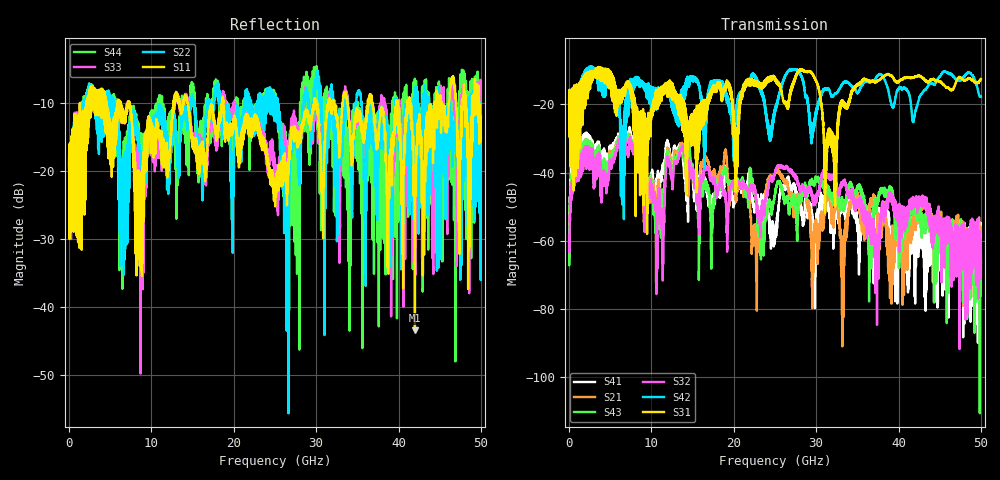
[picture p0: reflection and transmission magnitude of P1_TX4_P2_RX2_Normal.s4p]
!Keysight Technologies,N5225B,MY57041031,A.13.20.10
!Date: Friday, May 31, 2019 11:30:07
!Correction: S11(Full 4 Port(1,2,3,4))
!S12(Full 4 Port(1,2,3,4))
!S13(Full 4 Port(1,2,3,4))
!S14(Full 4 Port(1,2,3,4))
!S21(Full 4 Port(1,2,3,4))
!S22(Full 4 Port(1,2,3,4))
!S23(Full 4 Port(1,2,3,4))
!S24(Full 4 Port(1,2,3,4))
!S31(Full 4 Port(1,2,3,4))
!S32(Full 4 Port(1,2,3,4))
!S33(Full 4 Port(1,2,3,4))
!S34(Full 4 Port(1,2,3,4))
!S41(Full 4 Port(1,2,3,4))
!S42(Full 4 Port(1,2,3,4))
!S43(Full 4 Port(1,2,3,4))
!S44(Full 4 Port(1,2,3,4))
!S4P File: Measurements: <S11,S12,S13,S14>,
!<S21,S22,S23,S24>,
!<S31,S32,S33,S34>,
!<S41,S42,S43,S44>:
# Hz S  dB  R 50.0
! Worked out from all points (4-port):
!   5000 points, 10 MHz to 50 GHz, reference 50 ohm
!   strongest paths, dB at 10 MHz, 12.51 GHz, 25.01 GHz, 37.51 GHz, 50 GHz:
!     S31: -19.6, -17.9, -13.0, -13.1, -12.6
!     S42: -19.5, -15.9, -21.5, -11.4, -17.7
!     S32: -60.1, -41.7, -39.9, -62.8, -66.4
!     S43: -62.0, -40.3, -46.1, -48.8, -66.5
!     S21: -61.4, -38.6, -40.4, -55.7, -68.5
!     S41: -58.4, -35.8, -58.5, -51.1, -70.3
!   lowest |S11| = -43.4 dB at 41.99 GHz (marker M1), VSWR 1.01, Z = 50.7 - j0.157 ohm
!   |S11| at or under -10 dB: 7.334 GHz to 12.7 GHz (5.363 GHz wide, 53.5 % of centre); 14.44 GHz to 18.57 GHz (4.131 GHz wide, 25 % of centre); 18.74 GHz to 29.76 GHz (11.02 GHz wide, 45.4 % of centre)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
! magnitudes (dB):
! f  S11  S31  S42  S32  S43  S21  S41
! 10 MHz  -19.5  -19.6  -19.5  -60.1  -62.0  -61.4  -58.4
! 7.05 GHz  -11.0  -14.7  -22.4  -33.1  -29.1  -30.6  -28.9
! 10.47 GHz  -17.1  -17.5  -15.4  -48.0  -51.9  -52.2  -47.8
! 29.22 GHz  -12.6  -10.3  -25.2  -44.5  -43.0  -53.7  -50.9
! 32.24 GHz  -10.5  -35.9  -17.0  -42.5  -47.9  -51.3  -57.6
! 41.99 GHz  -43.4  -11.9  -22.7  -47.8  -49.7  -54.0  -55.4
! 50 GHz  -12.1  -12.6  -17.7  -66.4  -66.5  -68.5  -70.3
